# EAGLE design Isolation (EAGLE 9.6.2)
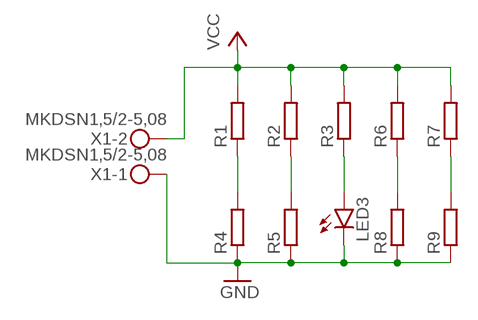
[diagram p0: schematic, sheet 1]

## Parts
LED3  LED5MM  [LED5MM]
R1  R-EU_0204/7  [0204/7]
R2  R-EU_0204/7  [0204/7]
R3  R-EU_0204/7  [0204/7]
R4  R-EU_0204/7  [0204/7]
R5  R-EU_0204/7  [0204/7]
R6  R-EU_0204/7  [0204/7]
R7  R-EU_0204/7  [0204/7]
R8  R-EU_0204/7  [0204/7]
R9  R-EU_0204/7  [0204/7]
X1  MKDSN1,5/2-5,08  [MKDSN1,5/2-5,08]

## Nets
GND: LED3.K(C) R4.1 R5.1 R8.1 R9.1 X1.1
N$1: R1.1 R4.2
N$2: R6.1 R8.2
N$3: R2.1 R5.2
N$4: LED3.A R3.1
N$5: R7.1 R9.2
VCC: R1.2 R2.2 R3.2 R6.2 R7.2 X1.2

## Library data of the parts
LED3 = led:LED: LED
R1-R9 = rcl:R-EU_: RESISTOR, European symbol; SPICEPREFIX: R
X1 = con-phoenix-508:MKDSN1,5/2-5,08: MKDSN 1,5/ 2-5,08 Printklemme

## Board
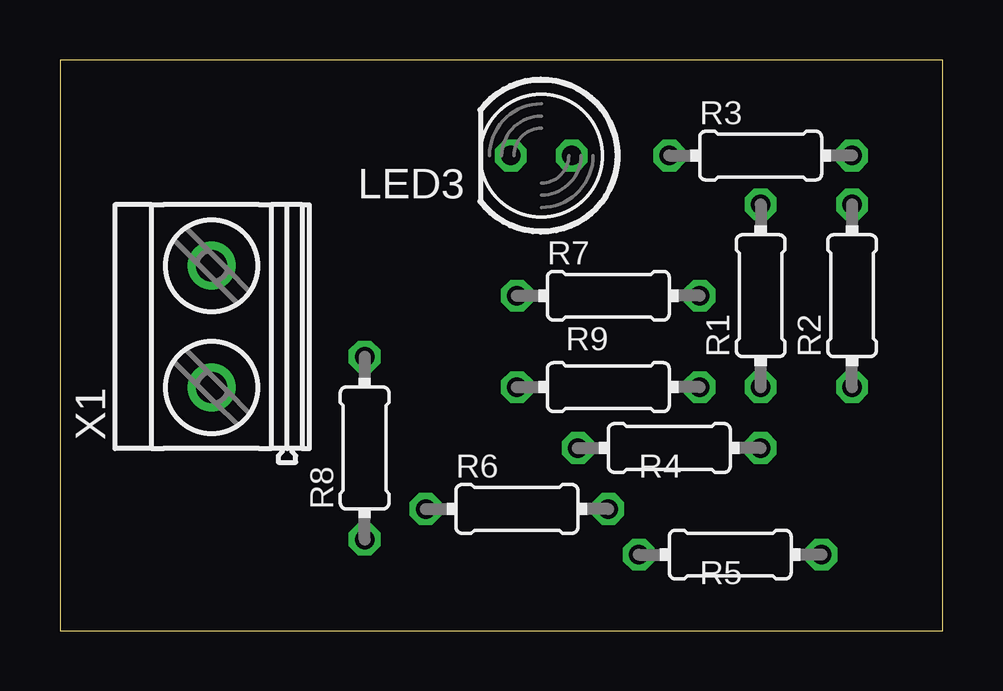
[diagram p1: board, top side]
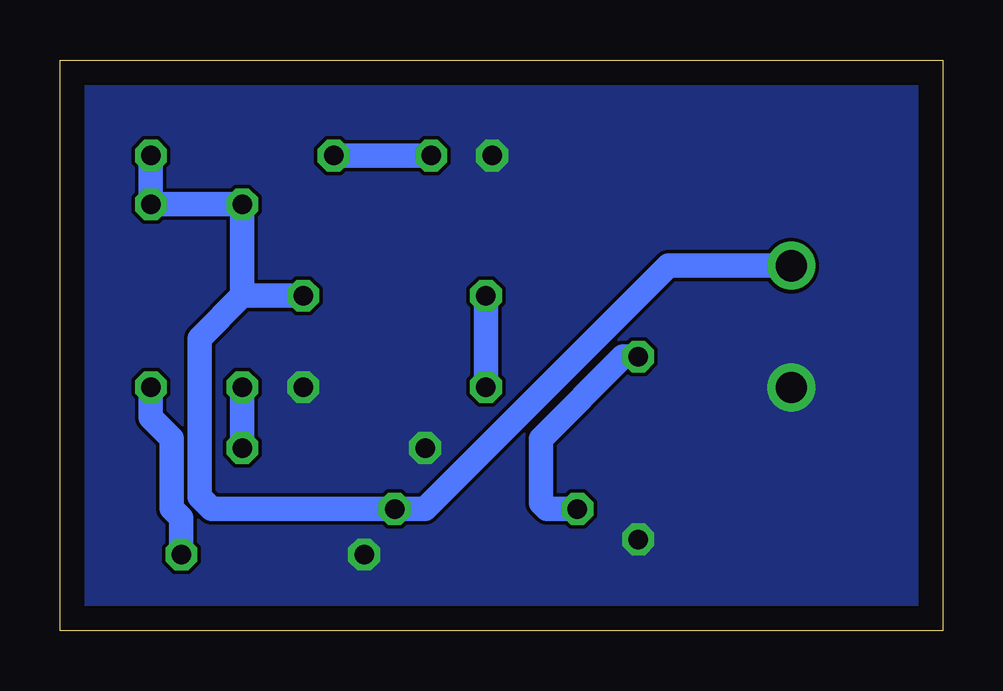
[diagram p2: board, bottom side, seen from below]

Size 36.81 x 23.8 mm. Coordinates in mm from the lower left corner, seen from the top.
Outline: 0,0 36.81,0 36.81,23.8 0,23.8 0,0
Copper layers (1*16): Top 0.035mm / dielectric 1.5mm / Bottom 0.035mm
Design rules "default": minimum track width 6mil, minimum drill 0.35mm, track to track 6mil, track to pad 6mil, pad to pad 6mil, via to via 6mil, smd to smd 6mil, copper to edge 40mil, drill to drill 6mil, minimum pad ring 10mil, minimum via ring 8mil, stop-mask expansion 4mil, vias tented up to drill 0mil, thermal gap 10mil

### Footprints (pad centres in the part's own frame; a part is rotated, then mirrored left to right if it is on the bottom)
LED5MM = drill 0.813 octagon: A -1.27,0; K 1.27,0
0204/7 = drill 0.813 octagon: 1 -3.81,0; 2 3.81,0
MKDSN1,5/2-5,08 = drill 1.3 pad 2: 1 -2.561,0.025; 2 2.519,0.025

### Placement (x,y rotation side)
LED3  20.07,19.81 180 top
R1  29.21,13.97 90 top
R2  33.02,13.97 90 top
R3  29.21,19.81 0 top
R4  25.4,7.62 0 top
R5  27.94,3.17 0 top
R6  19.05,5.08 0 top
R7  22.86,13.97 0 top
R8  12.7,7.62 90 top
R9  22.86,10.16 180 top
X1  6.35,12.7 90 top

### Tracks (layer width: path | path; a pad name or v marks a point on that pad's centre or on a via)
GND
  pour Bottom (isolate 0.1, rank 2, no thermals): 0,0 36.83,0 36.83,23.75 0,23.75
N$1
  Bottom 1.016: R1.1 R4.2
N$2
  Bottom 1.016: R8.2 13.34,11.43 16.76,8 16.76,5.33 16.51,5.08 R6.1
N$3
  Bottom 1.016: R2.1 33.02,8.89 32.16,8.03 32.16,5.1 31.75,4.7 R5.2
N$4
  Bottom 1.016: R3.1 LED3.A
N$5
  Bottom 1.016: R7.1 R9.2
VCC
  Bottom 1.016: R3.2 R2.2 R1.2 29.21,13.97 | 29.21,13.97 30.99,12.19 30.99,5.59 30.48,5.08 R6.2 21.59,5.08 11.45,15.22 X1.2 | 29.21,13.97 R7.2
